| IBIS file was generated by Viper version: 2025.10.06
[IBIS Ver]   6.0
[Comment Char]   |_char
[File Name]   c15x_c05x_48lqfp.ibs
[File Rev]   1.0
[Date]   Wed Oct 22 17:23:38 2025
[Source]   NXP Viper 2025.10.06
[Notes]
[Disclaimer] IMPORTANT NOTICE
  This information is provided on an AS IS basis and without warranty.
  IN NO EVENT SHALL NXP BE LIABLE FOR INCIDENTAL OR CONSEQUENTIAL
  DAMAGES ARISING FROM USE OF THIS INFORMATION. THIS DISCLAIMER OF
  WARRANTY EXTENDS TO THE USER OF THE INFORMATION, AND TO THEIR CUSTOMERS
  OR USERS OF PRODUCTS  AND IS IN LIEU OF ALL WARRANTIES WHETHER EXPRESS,
  IMPLIED, OR STATUTORY, INCLUDING IMPLIED WARRANTIES OF MERCHANTABILITY
  OR FITNESS FOR PARTICULAR PURPOSE.
  NXP does not represent or warrant that the information furnished
  hereunder is free of infringement of any third party patents,
  copyrights, trade secrets, or other intellectual property rights.
  NXP does not represent or warrant that the information is free of
  defect, or that it meets any particular standard, requirements or need
  of the user of the infomation or their customers.
  NXP reserves the right to change the information in this file
  without notice.
   http://www.nxp.com
[Copyright]   (C) Copyright NXP 2004 - 2025, All Rights Reserved.
|   C15x_C05x_48LQFP
[Component]   C15x_C05x_48LQFP
[Manufacturer]   NXP
[Package]
| variable   typ   min   max
R_pkg   0.21897   0.20464   0.24301
L_pkg   4.396e-09   3.463e-09   5.668e-09
C_pkg   2.263e-13   2.032e-13   2.586e-13
[Pin] signal_name   model_name   R_pin   L_pin   C_pin
1   P1_8   a_ip_io_3v_3p3v   0.22928   4.659e-09 2.454e-13
2   P1_9   a_ip_io_3v_3p3v   0.20837   4.297e-09 2.296e-13
3   P1_29   a_ip_io_3v_3p3v   0.20706   4.031e-09 2.207e-13
4   P1_30   a_ip_io_3v_3p3v   0.20752   3.774e-09 2.200e-13
5   P1_31   a_ip_io_3v_3p3v   0.21118   3.463e-09 2.168e-13
6   VSS   GND   NA   NA   NA
7   VDD_ANA   POWER   NA   NA   NA
8   VDD   POWER   NA   NA   NA
9   P2_0   a_ip_io_3v_3p3v   0.21124   3.515e-09 2.210e-13
10   P2_1   a_ip_io_3v_3p3v   0.21219   3.832e-09 2.333e-13
11   P2_2   a_ip_io_3v_3p3v   0.21775   4.167e-09 2.369e-13
12   P2_3   a_ip_io_3v_3p3v   0.22826   4.465e-09 2.433e-13
13   P2_6   a_ip_io_3v_3p3v   0.21856   4.532e-09 2.476e-13
14   P2_7   a_ip_io_3v_3p3v   0.21297   4.483e-09 2.402e-13
15   P2_12   a_ip_io_3v_3p3v   0.21041   4.457e-09 2.265e-13
16   P2_13   a_ip_io_3v_3p3v   0.21098   4.419e-09 2.193e-13
17   P2_16   a_ip_io_3v_3p3v   0.21487   4.453e-09 2.140e-13
18   P2_17   a_ip_io_3v_3p3v   0.23111   4.585e-09 2.069e-13
19   P2_20   a_ip_io_3v_3p3v   0.23173   4.598e-09 2.090e-13
20   P2_21   a_ip_io_3v_3p3v   0.21773   4.525e-09 2.181e-13
21   P2_27   a_ip_io_3v_3p3v   0.21648   4.547e-09 2.281e-13
22   P2_28   a_ip_io_3v_3p3v   0.21941   4.621e-09 2.383e-13
23   P3_31   a_ip_io_3v_3p3v   0.2272   4.823e-09 2.510e-13
24   P3_30   a_ip_io_3v_3p3v   0.23818   5.073e-09 2.586e-13
25   P3_29   a_ip_io_3v_3p3v   0.24301   4.941e-09 2.525e-13
26   P3_28   a_ip_io_3v_3p3v   0.21056   4.442e-09 2.278e-13
27   P3_27   a_ip_io_3v_3p3v   0.21213   4.390e-09 2.180e-13
28   P3_13   a_ip_io_3v_3p3v   0.21979   4.440e-09 2.189e-13
29   P3_12   a_ip_io_3v_3p3v   0.22127   4.404e-09 2.173e-13
30   P3_11   a_ip_io_3v_3p3v   0.23235   4.405e-09 2.060e-13
31   P3_10   a_ip_io_3v_3p3v   0.22803   4.229e-09 2.037e-13
32   P3_9   a_ip_io_3v_3p3v   0.21139   4.014e-09 2.125e-13
33   P3_8   a_ip_io_3v_3p3v   0.20846   3.986e-09 2.213e-13
34   P3_1   a_ip_io_3v_3p3v   0.20939   3.834e-09 2.291e-13
35   P3_0   a_ip_io_3v_3p3v   0.21379   3.680e-09 2.396e-13
36   VSS   GND   NA   NA   NA
37   VDD   POWER   NA   NA   NA
38   P0_0   a_ip_io_3v_3p3v   0.20603   3.533e-09 2.365e-13
39   P0_1   a_ip_io_3v_3p3v   0.20464   3.803e-09 2.274e-13
40   P0_2   a_ip_io_3v_3p3v   0.20584   4.020e-09 2.213e-13
41   P0_3   a_ip_io_3v_3p3v   0.21159   4.280e-09 2.108e-13
42   P0_6   a_ip_io_3v_3p3v   0.22871   4.576e-09 2.032e-13
43   P0_16   a_ip_io_3v_3p3v   0.23058   4.700e-09 2.059e-13
44   P0_17   a_ip_io_3v_3p3v   0.21957   4.772e-09 2.141e-13
45   P1_0   a_ip_io_3v_3p3v   0.21995   4.953e-09 2.222e-13
46   P1_1   a_ip_io_3v_3p3v   0.22456   5.198e-09 2.305e-13
47   P1_2   a_ip_io_3v_3p3v   0.23163   5.458e-09 2.407e-13
48   P1_3   a_ip_io_3v_3p3v   0.23981   5.668e-09 2.468e-13
[Pin Mapping]   pulldown_ref   pullup_ref
1   VSS   VDD
2   VSS   VDD
3   VSS   VDD
4   VSS   VDD
5   VSS   VDD
6   VSS   NC
7   NC   VDD_ANA
8   NC   VDD
9   VSS   VDD
10   VSS   VDD
11   VSS   VDD
12   VSS   VDD
13   VSS   VDD
14   VSS   VDD
15   VSS   VDD
16   VSS   VDD
17   VSS   VDD
18   VSS   VDD
19   VSS   VDD
20   VSS   VDD
21   VSS   VDD
22   VSS   VDD
23   VSS   VDD
24   VSS   VDD
25   VSS   VDD
26   VSS   VDD
27   VSS   VDD
28   VSS   VDD
29   VSS   VDD
30   VSS   VDD
31   VSS   VDD
32   VSS   VDD
33   VSS   VDD
34   VSS   VDD
35   VSS   VDD
36   VSS   NC
37   NC   VDD
38   VSS   VDD
39   VSS   VDD
40   VSS   VDD
41   VSS   VDD
42   VSS   VDD
43   VSS   VDD
44   VSS   VDD
45   VSS   VDD
46   VSS   VDD
47   VSS   VDD
48   VSS   VDD
|*   Model Selector   *
[Model Selector] a_ip_io_3v_3p3v
p_io_25mhz_ds0_sr0_3p3v_mio   dse=0 sre=0 25mhz
p_io_25mhz_ds0_sr1_3p3v_mio   dse=0 sre=1 25mhz
p_io_25mhz_ds1_sr0_3p3v_mio   dse=1 sre=0 25mhz
p_io_25mhz_ds1_sr1_3p3v_mio   dse=1 sre=1 25mhz
p_io_25mhz_r40_ds0_sr0_3p3v_mio   dse=0 sre=0 25mhz_r40
p_io_25mhz_r40_ds0_sr1_3p3v_mio   dse=0 sre=1 25mhz_r40
p_io_25mhz_r40_ds1_sr0_3p3v_mio   dse=1 sre=0 25mhz_r40
p_io_25mhz_r40_ds1_sr1_3p3v_mio   dse=1 sre=1 25mhz_r40
p_io_50mhz_ds0_sr0_3p3v_mio   dse=0 sre=0 50mhz
p_io_50mhz_ds0_sr1_3p3v_mio   dse=0 sre=1 50mhz
p_io_50mhz_ds1_sr0_3p3v_mio   dse=1 sre=0 50mhz
p_io_50mhz_ds1_sr1_3p3v_mio   dse=1 sre=1 50mhz
p_io_25mhz_cap_ds0_sr0_3p3v_mio   dse=0 sre=0 25mhz_cap
p_io_25mhz_cap_ds0_sr1_3p3v_mio   dse=0 sre=1 25mhz_cap
p_io_25mhz_cap_ds1_sr0_3p3v_mio   dse=1 sre=0 25mhz_cap
p_io_25mhz_cap_ds1_sr1_3p3v_mio   dse=1 sre=1 25mhz_cap
p_io_25mhz_2mux_ds0_sr0_3p3v_mio   dse=0 sre=0 25mhz_2mux
p_io_25mhz_2mux_ds0_sr1_3p3v_mio   dse=0 sre=1 25mhz_2mux
p_io_25mhz_2mux_ds1_sr0_3p3v_mio   dse=1 sre=0 25mhz_2mux
p_io_25mhz_2mux_ds1_sr1_3p3v_mio   dse=1 sre=1 25mhz_2mux
p_io_100mhz_ds0_sr0_3p3v_mio   dse=0 sre=0 100mhz
p_io_100mhz_ds0_sr1_3p3v_mio   dse=0 sre=1 100mhz
p_io_100mhz_ds1_sr0_3p3v_mio   dse=1 sre=0 100mhz
p_io_100mhz_ds1_sr1_3p3v_mio   dse=1 sre=1 100mhz
p_io_100mhz_weftd_ds0_sr0_3p3v_mio   dse=0 sre=0 100mhz
p_io_100mhz_weftd_ds0_sr1_3p3v_mio   dse=0 sre=1 100mhz
p_io_100mhz_weftd_ds1_sr0_3p3v_mio   dse=1 sre=0 100mhz
p_io_100mhz_weftd_ds1_sr1_3p3v_mio   dse=1 sre=1 100mhz
p_io_i2c_ds00_ds10_sr0_3p3v_mio   dse0=0 dse1=0 sre=0 i2c
p_io_i2c_ds00_ds10_sr1_3p3v_mio   dse0=0 dse1=0 sre=1 i2c
p_io_i2c_ds00_ds11_sr0_3p3v_mio   dse0=0 dse1=1 sre=0 i2c
p_io_i2c_ds00_ds11_sr1_3p3v_mio   dse0=0 dse1=1 sre=1 i2c
p_io_i2c_ds01_ds10_sr0_3p3v_mio   dse0=1 dse1=0 sre=0 i2c
p_io_i2c_ds01_ds10_sr1_3p3v_mio   dse0=1 dse1=0 sre=1 i2c
p_io_i2c_ds01_ds11_sr0_3p3v_mio   dse0=1 dse1=1 sre=0 i2c
p_io_i2c_ds01_ds11_sr1_3p3v_mio   dse0=1 dse1=1 sre=1 i2c
p_io_i2c_i2c1_3p3v_mio   ipp_i2c_lv=1 i2c
p_io_i2cfmp_ds00_ds10_sr0_3p3v_mio   dse0=0 dse1=0 sre=0 i2cfmp
p_io_i2cfmp_ds00_ds10_sr1_3p3v_mio   dse0=0 dse1=0 sre=1 i2cfmp
p_io_i2cfmp_ds00_ds11_sr0_3p3v_mio   dse0=0 dse1=1 sre=0 i2cfmp
p_io_i2cfmp_ds00_ds11_sr1_3p3v_mio   dse0=0 dse1=1 sre=1 i2cfmp
p_io_i2cfmp_ds01_ds10_sr0_3p3v_mio   dse0=1 dse1=0 sre=0 i2cfmp
p_io_i2cfmp_ds01_ds10_sr1_3p3v_mio   dse0=1 dse1=0 sre=1 i2cfmp
p_io_i2cfmp_ds01_ds11_sr0_3p3v_mio   dse0=1 dse1=1 sre=0 i2cfmp
p_io_i2cfmp_ds01_ds11_sr1_3p3v_mio   dse0=1 dse1=1 sre=1 i2cfmp
p_io_i2cfmp_i2c1_3p3v_mio   ipp_i2c_lv=1 i2cfmp
p_io_rst_3p3v_mio   rst
p_io_rst_rx1p8v_3p3v_mio   rst
p_io_aon_3p3v_mio   rst
| End [Component] C15x_C05x_48LQFP
| Models and submodels in the file (49): p_io_100mhz_ds0_sr0_3p3v_mio (I/O), p_io_100mhz_ds0_sr1_3p3v_mio (I/O), p_io_100mhz_ds1_sr0_3p3v_mio (I/O), p_io_100mhz_ds1_sr1_3p3v_mio (I/O), p_io_100mhz_weftd_ds0_sr0_3p3v_mio (I/O), p_io_100mhz_weftd_ds0_sr1_3p3v_mio (I/O), p_io_100mhz_weftd_ds1_sr0_3p3v_mio (I/O), p_io_100mhz_weftd_ds1_sr1_3p3v_mio (I/O), p_io_25mhz_2mux_ds0_sr0_3p3v_mio (I/O), p_io_25mhz_2mux_ds0_sr1_3p3v_mio (I/O), p_io_25mhz_2mux_ds1_sr0_3p3v_mio (I/O), p_io_25mhz_2mux_ds1_sr1_3p3v_mio (I/O), p_io_25mhz_cap_ds0_sr0_3p3v_mio (I/O), p_io_25mhz_cap_ds0_sr1_3p3v_mio (I/O), p_io_25mhz_cap_ds1_sr0_3p3v_mio (I/O), p_io_25mhz_cap_ds1_sr1_3p3v_mio (I/O), p_io_25mhz_ds0_sr0_3p3v_mio (I/O), p_io_25mhz_ds0_sr1_3p3v_mio (I/O), p_io_25mhz_ds1_sr0_3p3v_mio (I/O), p_io_25mhz_ds1_sr1_3p3v_mio (I/O), p_io_25mhz_r40_ds0_sr0_3p3v_mio (I/O), p_io_25mhz_r40_ds0_sr1_3p3v_mio (I/O), p_io_25mhz_r40_ds1_sr0_3p3v_mio (I/O), p_io_25mhz_r40_ds1_sr1_3p3v_mio (I/O), p_io_50mhz_ds0_sr0_3p3v_mio (I/O), p_io_50mhz_ds0_sr1_3p3v_mio (I/O), p_io_50mhz_ds1_sr0_3p3v_mio (I/O), p_io_50mhz_ds1_sr1_3p3v_mio (I/O), p_io_aon_3p3v_mio (I/O), p_io_i2c_ds00_ds10_sr0_3p3v_mio (I/O), p_io_i2c_ds00_ds10_sr1_3p3v_mio (I/O), p_io_i2c_ds00_ds11_sr0_3p3v_mio (I/O), p_io_i2c_ds00_ds11_sr1_3p3v_mio (I/O), p_io_i2c_ds01_ds10_sr0_3p3v_mio (I/O), p_io_i2c_ds01_ds10_sr1_3p3v_mio (I/O), p_io_i2c_ds01_ds11_sr0_3p3v_mio (I/O), p_io_i2c_ds01_ds11_sr1_3p3v_mio (I/O), p_io_i2c_i2c1_3p3v_mio (I/O), p_io_i2cfmp_ds00_ds10_sr0_3p3v_mio (I/O), p_io_i2cfmp_ds00_ds10_sr1_3p3v_mio (I/O), p_io_i2cfmp_ds00_ds11_sr0_3p3v_mio (I/O), p_io_i2cfmp_ds00_ds11_sr1_3p3v_mio (I/O), p_io_i2cfmp_ds01_ds10_sr0_3p3v_mio (I/O), p_io_i2cfmp_ds01_ds10_sr1_3p3v_mio (I/O), p_io_i2cfmp_ds01_ds11_sr0_3p3v_mio (I/O), p_io_i2cfmp_ds01_ds11_sr1_3p3v_mio (I/O), p_io_i2cfmp_i2c1_3p3v_mio (I/O), p_io_rst_3p3v_mio (I/O), p_io_rst_rx1p8v_3p3v_mio (I/O)
